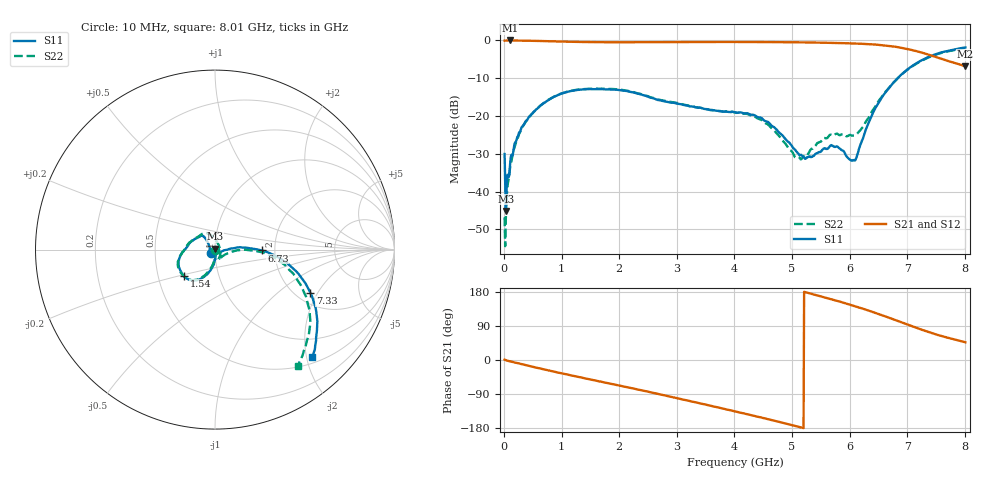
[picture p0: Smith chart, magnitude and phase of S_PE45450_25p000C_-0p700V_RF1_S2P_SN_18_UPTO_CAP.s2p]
! Device ID: PE45450
! Serial: 18
! Temp: 25.000C
! VCTRL: -0.700
! VSS: 0.000
! Control_Hi: 0.000
! Control_Lo: 0.000
! Logic State: LS_RF1
! Port 1: RF1
! Port 2: RF2
! ThroughPath:1-2
! IDD: 6.34836598e-009
! ISS: 2.59897833e-009
#  Hz  S  RI  R  50
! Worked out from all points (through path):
!   801 points, 10 MHz to 8.01 GHz, reference 50 ohm
!   highest |S21| = -0.02 dB at 100 MHz (marker M1); lowest = -6.9 dB at 8.01 GHz (marker M2)
!   group delay of S21, straight-line fit = 106 ps
!   lowest |S11| = -45.1 dB at 30 MHz (marker M3), VSWR 1.01, Z = 50.1 + j0.552 ohm
!   |S11| at or under -10 dB: start of sweep to 6.836 GHz
!   |S22| runs from -54.5 to -2.0 dB; largest |S21 - S12| = 0.025
!   S11 on the Smith chart (normalised r, x): 10 MHz: 0.95, -0.04; 1.54 GHz: 0.68, -0.21; 6.73 GHz: 1.70, -0.02; 7.33 GHz: 2.37, -1.74; 8.01 GHz: 0.62, -2.11
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1e7  -0.0229 -0.0215  0.991 0.0159  0.9973 -0.00812  -0.00215 -0.004
3e7  0.00061 0.00551  0.9946 -0.00767  0.9996 -0.0204  0.00261 -0.0031
6e7  0.00257 -0.0165  0.9962 -0.0326  0.9974 -0.0392  0.00231 -0.0114
1e8  0.00496 -0.0197  0.9959 -0.0604  0.9953 -0.0638  0.00192 -0.0197
2.4e8  -0.000942 -0.0538  0.9824 -0.147  0.9846 -0.1505  -0.00266 -0.0512
4.8e8  -0.0185 -0.1047  0.9424 -0.293  0.9433 -0.2939  -0.0231 -0.1032
8.7e8  -0.0781 -0.1622  0.8334 -0.497  0.8335 -0.4987  -0.0832 -0.1603
1.35e9  -0.1536 -0.1638  0.655 -0.6915  0.6551 -0.6909  -0.158 -0.1609
1.54e9  -0.1736 -0.1457  0.5748 -0.7544  0.5758 -0.7535  -0.1786 -0.1432
2.68e9  -0.1621 0.00701  0.00403 -0.9517  0.00482 -0.9512  -0.1643 0.00761
3.35e9  -0.1165 0.0553  -0.3664 -0.8816  -0.3648 -0.8815  -0.1152 0.0597
4.01e9  -0.0834 0.0742  -0.6805 -0.667  -0.6804 -0.6668  -0.0695 0.087
4.57e9  -0.0539 0.0646  -0.865 -0.3915  -0.8645 -0.391  -0.0176 0.0761
5.08e9  -0.0308 0.0137  -0.9397 -0.0823  -0.9388 -0.0824  0.0244 0.0139
5.35e9  -0.0258 -0.0129  -0.9322 0.0932  -0.9318 0.0931  0.0304 -0.0207
5.7e9  -0.019 -0.0357  -0.8681 0.3215  -0.8683 0.3205  0.0226 -0.0509
6.08e9  0.0177 -0.0191  -0.7234 0.5522  -0.7226 0.5521  0.0415 -0.0363
6.41e9  0.1116 0.0092  -0.5228 0.7138  -0.5225 0.7133  0.1216 -0.00442
6.68e9  0.2325 0.00143  -0.3132 0.7851  -0.3134 0.7842  0.234 -0.00944
6.73e9  0.2593 -0.00456  -0.2713 0.7911  -0.2723 0.7903  0.2608 -0.0142
7.33e9  0.532 -0.2417  0.1612 0.6426  0.1617 0.6422  0.5093 -0.2684
8.01e9  0.5427 -0.5971  0.3107 0.3301  0.3101 0.3309  0.4613 -0.6467
